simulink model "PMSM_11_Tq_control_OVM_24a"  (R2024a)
settings: Solver=VariableStepAuto  StartTime=0.0  StopTime=0.1  MaxStep=1e-6  RelTol=1e-6  AbsTol=1e-6
libraries: spsIGBTDiodeLib x6, spsVoltageMeasurementLib x4, spsCurrentMeasurementLib x3, spsControlledVoltageSourceLib x3, slpidlib x2, spsDCVoltageSourceLib x1, spsGroundLib x1, simulink x1, spsThreePhaseSeriesRLCBranchLib x1, spspowerguiLib x1

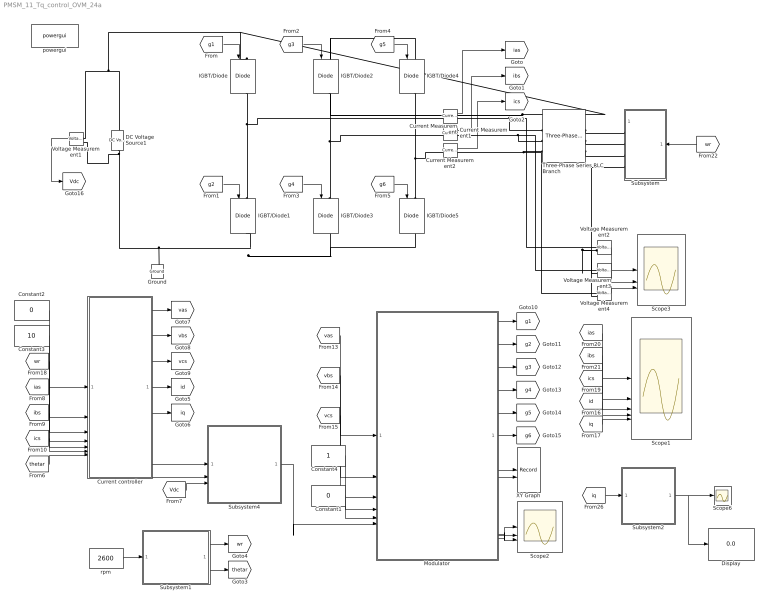
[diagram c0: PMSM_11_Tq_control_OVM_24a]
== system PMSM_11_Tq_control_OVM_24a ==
  Constant1 : Constant  Value=0
  Constant2 : Constant  Value=0
  Constant3 : Constant  Value=10
  Constant4 : Constant
  Current Measurement : spsCurrentMeasurementLib/Current Measurement  PhasorSimulation=off  OutputType=Complex  PSBequivalent=0
  Current Measurement1 : spsCurrentMeasurementLib/Current Measurement  PhasorSimulation=off  OutputType=Complex  PSBequivalent=0
  Current Measurement2 : spsCurrentMeasurementLib/Current Measurement  PhasorSimulation=off  OutputType=Complex  PSBequivalent=0
  Current controller : Subsystem
  DC Voltage Source1 : spsDCVoltageSourceLib/DC Voltage Source  Amplitude=200  Measurements=None
  Display : Display
  Ground : spsGroundLib/Ground  LConnTagsString=a
  IGBT/Diode{,1..5} (6 alike) : spsIGBTDiodeLib/IGBT//Diode  Ron=1e-3  Rs=1e5  Cs=inf  Measurements=on
  Modulator : Subsystem
  Scope1 : Scope  NumInputPorts=5
  Scope2 : Scope  NumInputPorts=3
  Scope3 : Scope  NumInputPorts=3
  Scope6 : Scope
  Subsystem : Subsystem
  Subsystem1 : Subsystem
  Subsystem2 : Subsystem
  Subsystem4 : Subsystem
  Three-Phase Series RLC Branch : spsThreePhaseSeriesRLCBranchLib/Three-Phase Series RLC Branch  LConnTagsString=A|B|C  RConnTagsString=A|B|C  BranchType=RL  Resistance=1  Inductance=2e-3  Capacitance=1e-6  Measurements=None
  Voltage Measurement{1..4} (4 alike) : spsVoltageMeasurementLib/Voltage Measurement  PhasorSimulation=off  OutputType=Complex  PSBequivalent=0
  XY Graph : Record  FileSettingsInternal="{\"entries\":[{\"content\":{\"excelSettings\":{\"content\":{},\"type\":\"Streamout.ExcelSettings\"},\"parquetSettings\":{\"content\":{},\"type\":\"Streamout.ParquetSettings\"}},\"type\":\"Streamout.FileSettingStorage\",\"uuid\":\"\"}],\"packageUris\":[\"http:\\/\\/schema.mathworks.com\\/mf0\\/streamout_blocks\\/R2020a\"],\"version\":\"1.0\"}"  Layout=[1 1]  SignalsInternal="{\"entries\":[{\"content\":{\"signals\":[{\"content\":{\"blockPath\":[],\"dimensions\":[1],\"domain\":\"\",\"lineColor\":\"#a2142f\",\"plots\":[ 1 ],\"port\":1,\"signalID\":1,\"signalName\":\"Modulator:7\"},\"type\":\"RecordBlkView.Signal\",\"uuid\":\"\"},{\"content\":{\"blockPath\":[],\"dimensions\":[1],\"domain\":\"\",\"lineColor\":\"#139fff\",\"plots\":[ 1 ],\"port\":2,\"signalID\":2,\"signalName\":\"Modulator:8\"},\"type\":\"RecordBlkView.Signal\",\"uuid\":\"\"}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"  VisualizationBindings="{\"xyplotplugin\":{\"info\":[{\"series\":[{\"bindingParametersList\":[{\"parameter\":\"X-Axis\",\"signalID\":1,\"signalName\":\"Modulator:7\"},{\"parameter\":\"Y-Axis\",\"signalID\":2,\"signalName\":\"Modulator:8\"}],\"seriesID\":0}],\"subplotID\":1}]}}"  CompatibilityTag=XY  st=0.0001
  powergui : spspowerguiLib/powergui  Priority=1  SimulationMode=Continuous  SampleTime=50e-6  frequency=60  Iterations=50  frequencyindice=0  Pbase=100e6  ErrMax=1e-4  UnitsV=kV  UnitsW=MW  buscounter=0  FunctionMessages=off  echomessages=off  EnableUseOfTLC=off  CurrentSourceSwitches=off  DisableSnubberDevices=off  DisableRonSwitches=off  DisableVfSwitches=off  DisplayEquations=off  AutomaticDiscreteSolvers=off  SolverType=Tustin/Backward Euler (TBE)  Interpol=off  ExternalGateDelay=off  methode=off  Ts=100  x0status=blocks  SPID=on  SwTol=0  HookPort=off  NonlinearTolerance=1e-4  nMaxIteration=100  ContinueOnMaxIteration=off  RestoreLinks=warning  ResistiveCurrentMeasurement=off  Frange=[0:2:500]  Ylog=off  Xlog=on  ShowGrid=off  save=off  variable=ZData  structure=0  ZoomFFT=off  StartTime=0.0  cycles=1  DisplayStyle=1  fundamental=60  FreqAxis=off  MaxFrequency=1000  frequencyindicesteady=1  RmsSteady=1  display=off
  rpm : Constant  Value=2600
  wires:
  [g1] -> IGBT/Diode/1
  [g2] -> IGBT/Diode1/1
  [g3] -> IGBT/Diode2/1
  [g4] -> IGBT/Diode3/1
  [g5] -> IGBT/Diode4/1
  [g6] -> IGBT/Diode5/1
  Current Measurement/1 -> [ias]
  Current Measurement1/1 -> [ibs]
  Current Measurement2/1 -> [ics]
  [id] -> Scope1/4
  [iq] -> Scope1/5
  [ias] -> Scope1/1
  [ics] -> Scope1/3
  [ibs] -> Scope1/2
  Voltage Measurement1/1 -> [Vdc]
  Voltage Measurement2/1 -> Scope3/1
  Voltage Measurement3/1 -> Scope3/2
  Voltage Measurement4/1 -> Scope3/3
  [wr] -> Subsystem/1(wr)
  Constant2/1 -> Current controller/1(id_ref)
  Constant3/1 -> Current controller/2(iq_ref)
  [wr] -> Current controller/3(wr)
  [ias] -> Current controller/4(ias)
  [ibs] -> Current controller/5(ibs)
  [ics] -> Current controller/6(ics)
  Current controller/1(vas) -> [vas]
  Current controller/2(vbs) -> [vbs]
  Current controller/3(vcs) -> [vcs]
  [thetar] -> Current controller/7(thetar)
  Current controller/4(id) -> [id]
  Current controller/5(iq) -> [iq]
  rpm/1 -> Subsystem1/1(rpm_ref)
  Subsystem1/1(wr) -> [wr]
  Subsystem1/2(thetar) -> [thetar]
  [vas] -> Modulator/1(vas)
  [vbs] -> Modulator/2(vbs)
  [vcs] -> Modulator/3(vcs)
  Constant4/1 -> Modulator/4(SVM_MODE)
  Constant1/1 -> Modulator/5(OVMgain)
  Modulator/1(g1) -> [g1]
  Modulator/2(g2) -> [g2]
  Modulator/3(g3) -> [g3]
  Modulator/4(g4) -> [g4]
  Modulator/5(g5) -> [g5]
  Modulator/6(g6) -> [g6]
  Subsystem2/1(Tq_avg) -> Scope6/1, Display/1
  [iq] -> Subsystem2/1(Iq)
  Modulator/7(Vds) -> XY Graph/1
  Modulator/8(Vqs) -> XY Graph/2
  Modulator/9(Van) -> Scope2/1
  Modulator/10(Vbn) -> Scope2/2
  Modulator/11(Vcn) -> Scope2/3
  Current controller/6(vds) -> Subsystem4/1(Vds)
  Current controller/7(vqs) -> Subsystem4/2(Vqs)
  [Vdc] -> Subsystem4/3(Vdc)
  Subsystem4/1(Flag_OVM) -> Modulator/6(Flag_OVM)
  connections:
  IGBT/Diode1/LConn1 -- Current Measurement/LConn1 -- IGBT/Diode/RConn1
  Voltage Measurement1/LConn1 -- IGBT/Diode4/LConn1 -- IGBT/Diode2/LConn1 -- IGBT/Diode/LConn1 -- DC Voltage Source1/RConn1
  DC Voltage Source1/LConn1 -- Voltage Measurement1/LConn2 -- IGBT/Diode3/RConn1 -- IGBT/Diode5/RConn1 -- IGBT/Diode1/RConn1 -- Ground/LConn1
  IGBT/Diode3/LConn1 -- Current Measurement1/LConn1 -- IGBT/Diode2/RConn1
  IGBT/Diode5/LConn1 -- Current Measurement2/LConn1 -- IGBT/Diode4/RConn1
  Three-Phase Series RLC Branch/RConn1 -- Subsystem/RConn1
  Three-Phase Series RLC Branch/RConn2 -- Subsystem/RConn2
  Three-Phase Series RLC Branch/RConn3 -- Subsystem/RConn3
  Current Measurement/RConn1 -- Voltage Measurement2/LConn1 -- Three-Phase Series RLC Branch/LConn1
  Current Measurement1/RConn1 -- Voltage Measurement3/LConn1 -- Three-Phase Series RLC Branch/LConn2
  Current Measurement2/RConn1 -- Voltage Measurement4/LConn1 -- Three-Phase Series RLC Branch/LConn3
  Voltage Measurement2/LConn2 -- Voltage Measurement4/LConn2 -- Voltage Measurement3/LConn2 -- Subsystem/RConn4

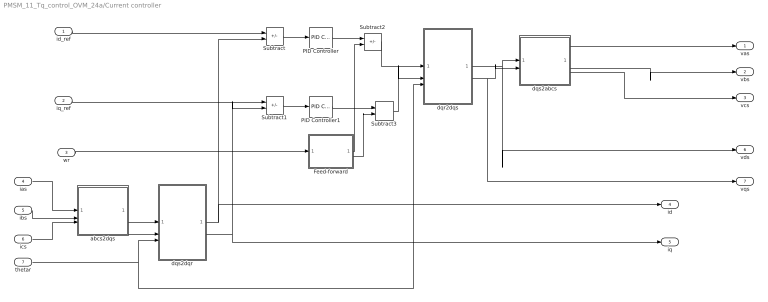
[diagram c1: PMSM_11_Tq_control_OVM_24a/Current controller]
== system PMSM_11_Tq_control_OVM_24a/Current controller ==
  id_ref : Inport
  iq_ref : Inport  Port=2
  wr : Inport  Port=3
  ias : Inport  Port=4
  ibs : Inport  Port=5
  ics : Inport  Port=6
  thetar : Inport  Port=7
  Feed-forward : Subsystem
  PID Controller : slpidlib/PID Controller  Controller=PI  Form=Parallel  TimeDomain=Continuous-time  UseExternalTs=off  SampleTime=-1  IntegratorMethod=Forward Euler  FilterMethod=Forward Euler  ControllerParametersSource=internal  P=2*pi*300*0.002  I=2*pi*300*1  UseKiTs=off  D=0  UseExternalDerivativeSource=off  N=100  UseFilter=on  TunerSelectOption=Transfer Function Based (PID Tuner App)  InitialConditionSource=internal  InitialConditionForIntegrator=0  InitialConditionForFilter=0  DifferentiatorICPrevScaledInput=0  ExternalReset=none  TrackingMode=off  Kt=1  LimitOutput=off  SatLimitsSource=internal  UpperSaturationLimit=inf  LowerSaturationLimit=-inf  LinearizeAsGain=on  AntiWindupMode=none  Kb=1  LimitIntegrator=off  UpperIntegratorSaturationLimit=inf  LowerIntegratorSaturationLimit=-inf  POutMin=[]  POutMax=[]  IOutMin=[]  IOutMax=[]  DOutMin=[]  DOutMax=[]  NOutMin=[]  NOutMax=[]  SumOutMin=[]  SumOutMax=[]  SaturationOutMin=[]  SaturationOutMax=[]  PParamMin=[]  PParamMax=[]  IParamMin=[]  IParamMax=[]  DParamMin=[]  DParamMax=[]  NParamMin=[]  NParamMax=[]  KbParamMin=[]  KbParamMax=[]  KtParamMin=[]  KtParamMax=[]  KbOutMin=[]  KbOutMax=[]  KtOutMin=[]  KtOutMax=[]  IntegratorOutMin=[]  IntegratorOutMax=[]  FilterOutMin=[]  FilterOutMax=[]  SumI1OutMin=[]  SumI1OutMax=[]  SumI2OutMin=[]  SumI2OutMax=[]  SumI3OutMin=[]  SumI3OutMax=[]  SumI4OutMin=[]  SumI4OutMax=[]  SumDOutMin=[]  SumDOutMax=[]  DifferentiatorOutMin=[]  DifferentiatorOutMax=[]  FilterDiffOutCoefMin=[]  FilterDiffOutCoefMax=[]  ReciprocalOutMin=[]  ReciprocalOutMax=[]  SumDenOutMin=[]  SumDenOutMax=[]  SumNumOutMin=[]  SumNumOutMax=[]  DivideOutMin=[]  DivideOutMax=[]  UdiffTsProdOutMin=[]  UdiffTsProdOutMax=[]  NTsProdOutMin=[]  NTsProdOutMax=[]  UintegralTsProdOutMin=[]  UintegralTsProdOutMax=[]  UngainTsProdOutMin=[]  UngainTsProdOutMax=[]  ClampingZeroOutDataTypeStr=Inherit: Inherit via back propagation  ClampingZeroOutMin=[]  ClampingZeroOutMax=[]  FilterDenConstantOutDataTypeStr=Inherit: Inherit via back propagation  FilterDenConstantOutMin=[]  FilterDenConstantOutMax=[]  PCopyOutDataTypeStr=Inherit: Inherit via back propagation  PCopyOutMin=[]  PCopyOutMax=[]  NCopyOutDataTypeStr=Inherit: Inherit via back propagation  NCopyOutMin=[]  NCopyOutMax=[]  IntegratorContinuousStateAttributes=''  IntegratorStateMustResolveToSignalObject=off  IntegratorRTWStateStorageClass=Auto  FilterContinuousStateAttributes=''  FilterStateMustResolveToSignalObject=off  FilterRTWStateStorageClass=Auto  ParallelPVariant=InternalParameters  IdealPVariant=Disabled  IVariant=InternalParameters  DVariant=Disabled  IntegratorVariant=Continuous  SatVariant=Disabled  AWVariant=Passthrough  PCopyVariant=Disabled  TRVariant=Disabled  FdbkBlocksVariant=Forward  IdealPFdbkVariant=Disabled  SatFdbkVariant=Disabled  DerivativeFilterVariant=Disabled  NVariant=Disabled  NCopyVariant=Disabled_SignalSpec  FilterICVariant=Disabled  IntegratorICVariant=InternalICs  ExternalResetVariant=Disabled  TRSumVariant=Passthrough  SumFdbkVariant=Disabled  SumVariant=Sum_PI  TsampFilterVariant=InternalTs  TsampNgainVariant=Passthrough  TsampIntegralVariant=Disabled_SignalSpec  ExternalSaturationOutDataTypeStr=Inherit: Same as second input  DerivativeSourceVariant=Disabled
  PID Controller1 : slpidlib/PID Controller  Controller=PI  Form=Parallel  TimeDomain=Continuous-time  UseExternalTs=off  SampleTime=-1  IntegratorMethod=Forward Euler  FilterMethod=Forward Euler  ControllerParametersSource=internal  P=2*pi*300*0.002  I=2*pi*300*1  UseKiTs=off  D=0  UseExternalDerivativeSource=off  N=100  UseFilter=on  TunerSelectOption=Transfer Function Based (PID Tuner App)  InitialConditionSource=internal  InitialConditionForIntegrator=0  InitialConditionForFilter=0  DifferentiatorICPrevScaledInput=0  ExternalReset=none  TrackingMode=off  Kt=1  LimitOutput=off  SatLimitsSource=internal  UpperSaturationLimit=inf  LowerSaturationLimit=-inf  LinearizeAsGain=on  AntiWindupMode=none  Kb=1  LimitIntegrator=off  UpperIntegratorSaturationLimit=inf  LowerIntegratorSaturationLimit=-inf  POutMin=[]  POutMax=[]  IOutMin=[]  IOutMax=[]  DOutMin=[]  DOutMax=[]  NOutMin=[]  NOutMax=[]  SumOutMin=[]  SumOutMax=[]  SaturationOutMin=[]  SaturationOutMax=[]  PParamMin=[]  PParamMax=[]  IParamMin=[]  IParamMax=[]  DParamMin=[]  DParamMax=[]  NParamMin=[]  NParamMax=[]  KbParamMin=[]  KbParamMax=[]  KtParamMin=[]  KtParamMax=[]  KbOutMin=[]  KbOutMax=[]  KtOutMin=[]  KtOutMax=[]  IntegratorOutMin=[]  IntegratorOutMax=[]  FilterOutMin=[]  FilterOutMax=[]  SumI1OutMin=[]  SumI1OutMax=[]  SumI2OutMin=[]  SumI2OutMax=[]  SumI3OutMin=[]  SumI3OutMax=[]  SumI4OutMin=[]  SumI4OutMax=[]  SumDOutMin=[]  SumDOutMax=[]  DifferentiatorOutMin=[]  DifferentiatorOutMax=[]  FilterDiffOutCoefMin=[]  FilterDiffOutCoefMax=[]  ReciprocalOutMin=[]  ReciprocalOutMax=[]  SumDenOutMin=[]  SumDenOutMax=[]  SumNumOutMin=[]  SumNumOutMax=[]  DivideOutMin=[]  DivideOutMax=[]  UdiffTsProdOutMin=[]  UdiffTsProdOutMax=[]  NTsProdOutMin=[]  NTsProdOutMax=[]  UintegralTsProdOutMin=[]  UintegralTsProdOutMax=[]  UngainTsProdOutMin=[]  UngainTsProdOutMax=[]  ClampingZeroOutDataTypeStr=Inherit: Inherit via back propagation  ClampingZeroOutMin=[]  ClampingZeroOutMax=[]  FilterDenConstantOutDataTypeStr=Inherit: Inherit via back propagation  FilterDenConstantOutMin=[]  FilterDenConstantOutMax=[]  PCopyOutDataTypeStr=Inherit: Inherit via back propagation  PCopyOutMin=[]  PCopyOutMax=[]  NCopyOutDataTypeStr=Inherit: Inherit via back propagation  NCopyOutMin=[]  NCopyOutMax=[]  IntegratorContinuousStateAttributes=''  IntegratorStateMustResolveToSignalObject=off  IntegratorRTWStateStorageClass=Auto  FilterContinuousStateAttributes=''  FilterStateMustResolveToSignalObject=off  FilterRTWStateStorageClass=Auto  ParallelPVariant=InternalParameters  IdealPVariant=Disabled  IVariant=InternalParameters  DVariant=Disabled  IntegratorVariant=Continuous  SatVariant=Disabled  AWVariant=Passthrough  PCopyVariant=Disabled  TRVariant=Disabled  FdbkBlocksVariant=Forward  IdealPFdbkVariant=Disabled  SatFdbkVariant=Disabled  DerivativeFilterVariant=Disabled  NVariant=Disabled  NCopyVariant=Disabled_SignalSpec  FilterICVariant=Disabled  IntegratorICVariant=InternalICs  ExternalResetVariant=Disabled  TRSumVariant=Passthrough  SumFdbkVariant=Disabled  SumVariant=Sum_PI  TsampFilterVariant=InternalTs  TsampNgainVariant=Passthrough  TsampIntegralVariant=Disabled_SignalSpec  ExternalSaturationOutDataTypeStr=Inherit: Same as second input  DerivativeSourceVariant=Disabled
  Subtract : Sum  Inputs=+-
  Subtract1 : Sum  Inputs=+-
  Subtract2 : Sum  Inputs=+-
  Subtract3 : Sum
  abcs2dqs : Subsystem
  dqr2dqs : Subsystem
  dqs2abcs : Subsystem
  dqs2dqr : Subsystem
  vas : Outport  VectorParamsAs1DForOutWhenUnconnected=off
  vbs : Outport  Port=2  VectorParamsAs1DForOutWhenUnconnected=off
  vcs : Outport  Port=3  VectorParamsAs1DForOutWhenUnconnected=off
  id : Outport  Port=4  VectorParamsAs1DForOutWhenUnconnected=off
  iq : Outport  Port=5  VectorParamsAs1DForOutWhenUnconnected=off
  vds : Outport  Port=6  VectorParamsAs1DForOutWhenUnconnected=off
  vqs : Outport  Port=7  VectorParamsAs1DForOutWhenUnconnected=off
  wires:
  thetar/1 -> dqs2dqr/3(thetar), dqr2dqs/3(thetar)
  dqr2dqs/2(qs) -> vqs/1, dqs2abcs/2(qs)
  dqr2dqs/1(ds) -> vds/1, dqs2abcs/1(ds)
  dqs2dqr/1(dr) -> id/1, Subtract/2
  abcs2dqs/1(ds) -> dqs2dqr/1(ds)
  Subtract/1 -> PID Controller/1
  dqs2dqr/2(qr) -> Subtract1/2, iq/1
  Subtract1/1 -> PID Controller1/1
  Feed-forward/1(Edr) -> Subtract2/2
  PID Controller1/1 -> Subtract3/1
  Subtract3/1 -> dqr2dqs/2(qr)
  abcs2dqs/2(qs) -> dqs2dqr/2(qs)
  ics/1 -> abcs2dqs/3(cs)
  Subtract2/1 -> dqr2dqs/1(dr)
  Feed-forward/2(Eqr) -> Subtract3/2
  PID Controller/1 -> Subtract2/1
  wr/1 -> Feed-forward/1(wr)
  iq_ref/1 -> Subtract1/1
  id_ref/1 -> Subtract/1
  ibs/1 -> abcs2dqs/2(bs)
  ias/1 -> abcs2dqs/1(as)
  dqs2abcs/1(as) -> vas/1
  dqs2abcs/2(bs) -> vbs/1
  dqs2abcs/3(cs) -> vcs/1

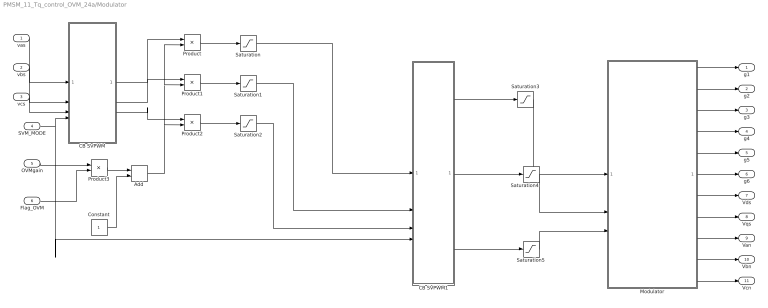
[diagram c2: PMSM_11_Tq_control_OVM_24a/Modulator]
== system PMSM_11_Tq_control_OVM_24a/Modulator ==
  vas : Inport
  vbs : Inport  Port=2
  vcs : Inport  Port=3
  SVM_MODE : Inport  Port=4
  OVMgain : Inport  Port=5
  Flag_OVM : Inport  Port=6
  Add : Sum
  CB SVPWM : Subsystem
  CB SVPWM1 : Subsystem
  Constant : Constant
  Modulator : Subsystem
  Product{,1..3} (4 alike) : Product
  Saturation{,1..5} (6 alike) : Saturate  UpperLimit=100  LowerLimit=-100
  g1 : Outport  VectorParamsAs1DForOutWhenUnconnected=off
  g2 : Outport  Port=2  VectorParamsAs1DForOutWhenUnconnected=off
  g3 : Outport  Port=3  VectorParamsAs1DForOutWhenUnconnected=off
  g4 : Outport  Port=4  VectorParamsAs1DForOutWhenUnconnected=off
  g5 : Outport  Port=5  VectorParamsAs1DForOutWhenUnconnected=off
  g6 : Outport  Port=6  VectorParamsAs1DForOutWhenUnconnected=off
  Vds : Outport  Port=7  VectorParamsAs1DForOutWhenUnconnected=off
  Vqs : Outport  Port=8  VectorParamsAs1DForOutWhenUnconnected=off
  Van : Outport  Port=9  VectorParamsAs1DForOutWhenUnconnected=off
  Vbn : Outport  Port=10  VectorParamsAs1DForOutWhenUnconnected=off
  Vcn : Outport  Port=11  VectorParamsAs1DForOutWhenUnconnected=off
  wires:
  CB SVPWM1/3(vcn) -> Saturation5/1
  vcs/1 -> CB SVPWM/3(vcs)
  Modulator/2(g2) -> g2/1
  CB SVPWM1/1(van) -> Saturation3/1
  Modulator/9(Van_inv) -> Van/1
  CB SVPWM1/2(vbn) -> Saturation4/1
  Modulator/5(g5) -> g5/1
  Modulator/4(g4) -> g4/1
  SVM_MODE/1 -> CB SVPWM1/4(SVM), CB SVPWM/4(SVM)
  vbs/1 -> CB SVPWM/2(vbs)
  Modulator/1(g1) -> g1/1
  Modulator/8(Vqs_stator) -> Vqs/1
  Modulator/6(g6) -> g6/1
  vas/1 -> CB SVPWM/1(vas)
  Modulator/10(Vbn_inv) -> Vbn/1
  Modulator/11(Vcn_inv) -> Vcn/1
  Modulator/7(Vds_stator) -> Vds/1
  Modulator/3(g3) -> g3/1
  Saturation3/1 -> Modulator/1(van)
  Saturation4/1 -> Modulator/2(vbn)
  Saturation5/1 -> Modulator/3(vcn)
  Product/1 -> Saturation/1
  Product1/1 -> Saturation1/1
  Product2/1 -> Saturation2/1
  CB SVPWM/1(van) -> Product/1
  CB SVPWM/3(vcn) -> Product2/1
  CB SVPWM/2(vbn) -> Product1/1
  OVMgain/1 -> Product3/1
  Flag_OVM/1 -> Product3/2
  Product3/1 -> Add/1
  Add/1 -> Product2/2, Product1/2, Product/2
  Constant/1 -> Add/2
  Saturation/1 -> CB SVPWM1/1(vas)
  Saturation1/1 -> CB SVPWM1/2(vbs)
  Saturation2/1 -> CB SVPWM1/3(vcs)

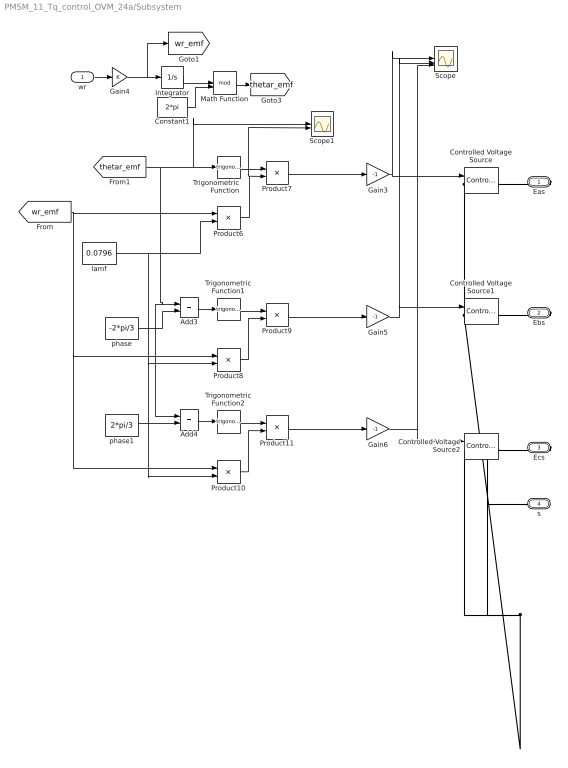
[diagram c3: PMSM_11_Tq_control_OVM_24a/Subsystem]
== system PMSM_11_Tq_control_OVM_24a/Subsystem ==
  wr : Inport
  Add3 : Sum
  Add4 : Sum
  Constant1 : Constant  Value=2*pi
  Controlled Voltage Source : spsControlledVoltageSourceLib/Controlled Voltage Source  Initialize=on  Source_Type=AC  Amplitude=0  Phase=0  Frequency=0  Measurements=None
  Controlled Voltage Source1 : spsControlledVoltageSourceLib/Controlled Voltage Source  Initialize=on  Source_Type=AC  Amplitude=0  Phase=0  Frequency=0  Measurements=None
  Controlled Voltage Source2 : spsControlledVoltageSourceLib/Controlled Voltage Source  Initialize=on  Source_Type=AC  Amplitude=0  Phase=0  Frequency=0  Measurements=None
  Gain3 : Gain  Gain=-1
  Gain4 : Gain
  Gain5 : Gain  Gain=-1
  Gain6 : Gain  Gain=-1
  Integrator : Integrator
  Math Function : Math  Operator=mod  SignedPower=on
  Product{6..11} (6 alike) : Product
  Scope : Scope  NumInputPorts=3
  Scope1 : Scope  NumInputPorts=2
  Trigonometric Function : Trigonometry
  Trigonometric Function1 : Trigonometry
  Trigonometric Function2 : Trigonometry
  lamf : Constant  Value=0.0796
  phase : Constant  Value=-2*pi/3
  phase1 : Constant  Value=2*pi/3
  Eas : PMIOPort  Side=Right
  Ebs : PMIOPort  Port=2  Side=Right
  Ecs : PMIOPort  Port=3  Side=Right
  s : PMIOPort  Port=4  Side=Right
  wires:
  Integrator/1 -> Math Function/1
  Constant1/1 -> Math Function/2
  Math Function/1 -> [thetar_emf]
  wr/1 -> Gain4/1
  Trigonometric Function/1 -> Product7/1
  Product6/1 -> Scope1/2, Product7/2
  Gain4/1 -> [wr_emf], Integrator/1
  Product7/1 -> Gain3/1
  Product9/1 -> Gain5/1
  Product8/1 -> Product9/2
  Trigonometric Function1/1 -> Product9/1
  [thetar_emf] -> Add4/1, Add3/1, Scope1/1, Trigonometric Function/1
  Add3/1 -> Trigonometric Function1/1
  phase/1 -> Add3/2
  Gain5/1 -> Controlled Voltage Source1/1, Scope/2
  Gain3/1 -> Controlled Voltage Source/1, Scope/1
  phase1/1 -> Add4/2
  Add4/1 -> Trigonometric Function2/1
  [wr_emf] -> Product10/1, Product8/1, Product6/1
  Trigonometric Function2/1 -> Product11/1
  Product10/1 -> Product11/2
  Product11/1 -> Gain6/1
  lamf/1 -> Product8/2, Product10/2, Product6/2
  Gain6/1 -> Controlled Voltage Source2/1, Scope/3
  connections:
  Eas/RConn1 -- Controlled Voltage Source/RConn1
  Ebs/RConn1 -- Controlled Voltage Source1/RConn1
  Ecs/RConn1 -- Controlled Voltage Source2/RConn1
  Controlled Voltage Source/LConn1 -- s/RConn1 -- Controlled Voltage Source2/LConn1 -- Controlled Voltage Source1/LConn1

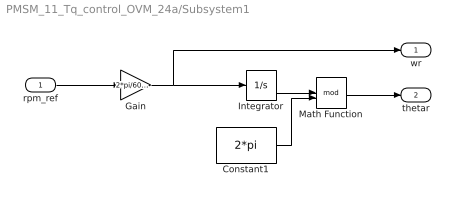
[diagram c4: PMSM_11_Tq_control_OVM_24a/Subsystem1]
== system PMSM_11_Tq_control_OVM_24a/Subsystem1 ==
  rpm_ref : Inport
  Constant1 : Constant  Value=2*pi
  Gain : Gain  Gain=2*pi/60*4
  Integrator : Integrator
  Math Function : Math  Operator=mod  SignedPower=on
  wr : Outport  VectorParamsAs1DForOutWhenUnconnected=off
  thetar : Outport  Port=2  VectorParamsAs1DForOutWhenUnconnected=off
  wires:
  Math Function/1 -> thetar/1
  Integrator/1 -> Math Function/1
  Gain/1 -> wr/1, Integrator/1
  rpm_ref/1 -> Gain/1
  Constant1/1 -> Math Function/2

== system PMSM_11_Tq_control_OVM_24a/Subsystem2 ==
  Iq : Inport
  Tq_constant : Gain  Gain=3/4*4*0.0796
  Transfer Fcn : TransferFcn  Numerator=[2*pi*50]  Denominator=[1 2*pi*50]
  Tq_avg : Outport  VectorParamsAs1DForOutWhenUnconnected=off
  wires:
  Transfer Fcn/1 -> Tq_avg/1
  Iq/1 -> Tq_constant/1
  Tq_constant/1 -> Transfer Fcn/1

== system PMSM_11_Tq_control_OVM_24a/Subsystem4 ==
  Vds : Inport
  Vqs : Inport  Port=2
  Vdc : Inport  Port=3
  Gain : Gain  Gain=1/sqrt(3)
  Relational Operator : RelationalOperator  Operator=>  OutDataTypeStr=boolean  RndMeth=Simplest
  Subsystem3 : Subsystem
  Flag_OVM : Outport
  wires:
  Subsystem3/1(Out1) -> Relational Operator/1
  Vdc/1 -> Gain/1
  Relational Operator/1 -> Flag_OVM/1
  Vds/1 -> Subsystem3/1(In1)
  Gain/1 -> Relational Operator/2
  Vqs/1 -> Subsystem3/2(In2)

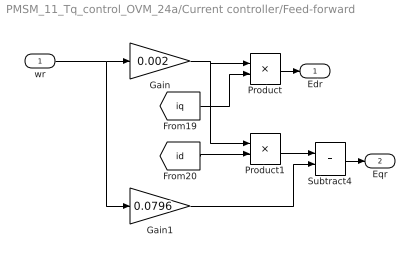
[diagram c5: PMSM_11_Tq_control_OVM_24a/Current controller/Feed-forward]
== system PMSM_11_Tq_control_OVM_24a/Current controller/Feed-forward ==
  wr : Inport
  Gain : Gain  Gain=0.002
  Gain1 : Gain  Gain=0.0796
  Product : Product
  Product1 : Product
  Subtract4 : Sum
  Edr : Outport  VectorParamsAs1DForOutWhenUnconnected=off
  Eqr : Outport  Port=2  VectorParamsAs1DForOutWhenUnconnected=off
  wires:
  Gain/1 -> Product1/1, Product/1
  Gain1/1 -> Subtract4/2
  [id] -> Product1/2
  wr/1 -> Gain1/1, Gain/1
  Product1/1 -> Subtract4/1
  [iq] -> Product/2
  Product/1 -> Edr/1
  Subtract4/1 -> Eqr/1

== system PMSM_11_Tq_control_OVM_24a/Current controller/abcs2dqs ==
  as : Inport
  bs : Inport  Port=2
  cs : Inport  Port=3
  Gain : Gain  Gain=1/sqrt(3)
  Subtract : Sum  Inputs=+-
  ds : Outport  VectorParamsAs1DForOutWhenUnconnected=off
  qs : Outport  Port=2  VectorParamsAs1DForOutWhenUnconnected=off
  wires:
  Subtract/1 -> Gain/1
  Gain/1 -> qs/1
  bs/1 -> Subtract/1
  cs/1 -> Subtract/2
  as/1 -> ds/1

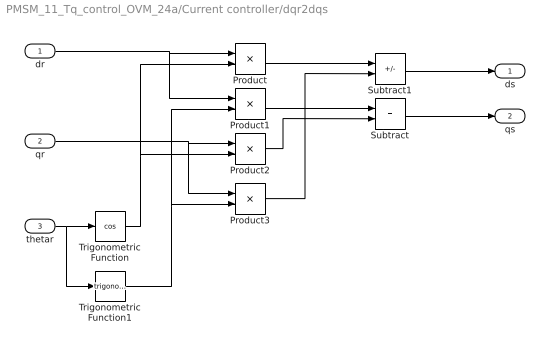
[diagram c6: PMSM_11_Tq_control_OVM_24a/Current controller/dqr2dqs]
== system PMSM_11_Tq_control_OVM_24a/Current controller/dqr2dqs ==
  dr : Inport
  qr : Inport  Port=2
  thetar : Inport  Port=3
  Product{,1..3} (4 alike) : Product
  Subtract : Sum
  Subtract1 : Sum  Inputs=+-
  Trigonometric Function : Trigonometry  Operator=cos
  Trigonometric Function1 : Trigonometry
  ds : Outport  VectorParamsAs1DForOutWhenUnconnected=off
  qs : Outport  Port=2  VectorParamsAs1DForOutWhenUnconnected=off
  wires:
  Subtract1/1 -> ds/1
  Product2/1 -> Subtract/2
  Product1/1 -> Subtract/1
  Product3/1 -> Subtract1/2
  Product/1 -> Subtract1/1
  qr/1 -> Product2/1, Product3/1
  Trigonometric Function1/1 -> Product1/2, Product3/2
  Trigonometric Function/1 -> Product/2, Product2/2
  dr/1 -> Product/1, Product1/1
  thetar/1 -> Trigonometric Function/1, Trigonometric Function1/1
  Subtract/1 -> qs/1

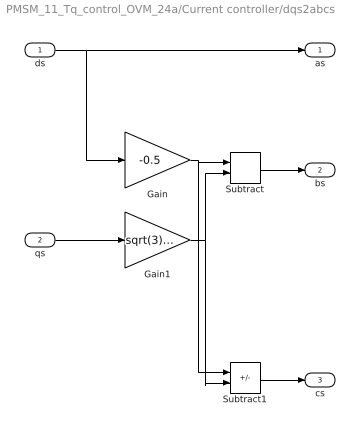
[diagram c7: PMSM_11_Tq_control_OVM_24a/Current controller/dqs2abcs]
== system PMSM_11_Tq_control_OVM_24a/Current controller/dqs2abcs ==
  ds : Inport
  qs : Inport  Port=2
  Gain : Gain  Gain=-0.5
  Gain1 : Gain  Gain=sqrt(3)/2
  Subtract : Sum
  Subtract1 : Sum  Inputs=+-
  as : Outport  VectorParamsAs1DForOutWhenUnconnected=off
  bs : Outport  Port=2  VectorParamsAs1DForOutWhenUnconnected=off
  cs : Outport  Port=3  VectorParamsAs1DForOutWhenUnconnected=off
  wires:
  ds/1 -> Gain/1, as/1
  Gain/1 -> Subtract1/1, Subtract/1
  qs/1 -> Gain1/1
  Gain1/1 -> Subtract/2, Subtract1/2
  Subtract/1 -> bs/1
  Subtract1/1 -> cs/1

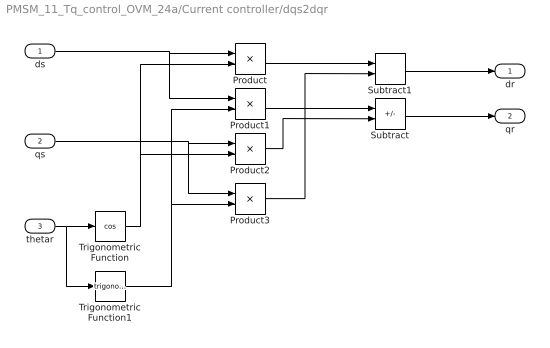
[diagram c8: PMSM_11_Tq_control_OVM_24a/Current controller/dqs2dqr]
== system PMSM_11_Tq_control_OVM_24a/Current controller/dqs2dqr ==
  ds : Inport
  qs : Inport  Port=2
  thetar : Inport  Port=3
  Product{,1..3} (4 alike) : Product
  Subtract : Sum  Inputs=-+
  Subtract1 : Sum
  Trigonometric Function : Trigonometry  Operator=cos
  Trigonometric Function1 : Trigonometry
  dr : Outport  VectorParamsAs1DForOutWhenUnconnected=off
  qr : Outport  Port=2  VectorParamsAs1DForOutWhenUnconnected=off
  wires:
  Subtract/1 -> qr/1
  thetar/1 -> Trigonometric Function1/1, Trigonometric Function/1
  ds/1 -> Product1/1, Product/1
  Trigonometric Function/1 -> Product2/2, Product/2
  Trigonometric Function1/1 -> Product3/2, Product1/2
  qs/1 -> Product3/1, Product2/1
  Product/1 -> Subtract1/1
  Product3/1 -> Subtract1/2
  Product1/1 -> Subtract/1
  Product2/1 -> Subtract/2
  Subtract1/1 -> dr/1

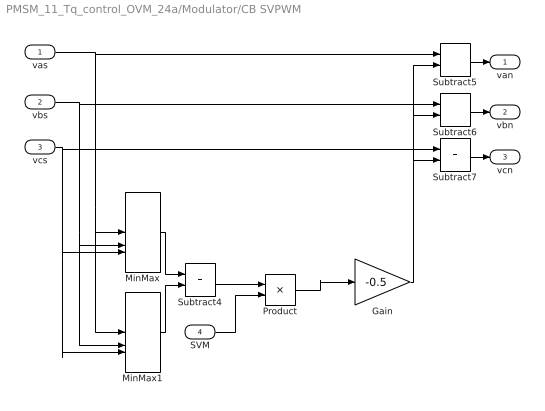
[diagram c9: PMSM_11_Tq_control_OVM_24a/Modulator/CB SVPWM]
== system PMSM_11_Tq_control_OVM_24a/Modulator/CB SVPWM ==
  vas : Inport
  vbs : Inport  Port=2
  vcs : Inport  Port=3
  SVM : Inport  Port=4
  Gain : Gain  Gain=-0.5
  MinMax : MinMax  Function=max  Inputs=3
  MinMax1 : MinMax  Inputs=3
  Product : Product
  Subtract{4..7} (4 alike) : Sum
  van : Outport  VectorParamsAs1DForOutWhenUnconnected=off
  vbn : Outport  Port=2  VectorParamsAs1DForOutWhenUnconnected=off
  vcn : Outport  Port=3  VectorParamsAs1DForOutWhenUnconnected=off
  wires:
  MinMax/1 -> Subtract4/1
  MinMax1/1 -> Subtract4/2
  vcs/1 -> MinMax1/3, MinMax/3, Subtract7/1
  Subtract6/1 -> vbn/1
  vbs/1 -> MinMax1/2, MinMax/2, Subtract6/1
  Subtract5/1 -> van/1
  Gain/1 -> Subtract6/2, Subtract5/2, Subtract7/2
  vas/1 -> MinMax1/1, MinMax/1, Subtract5/1
  Subtract7/1 -> vcn/1
  Subtract4/1 -> Product/1
  Product/1 -> Gain/1
  SVM/1 -> Product/2

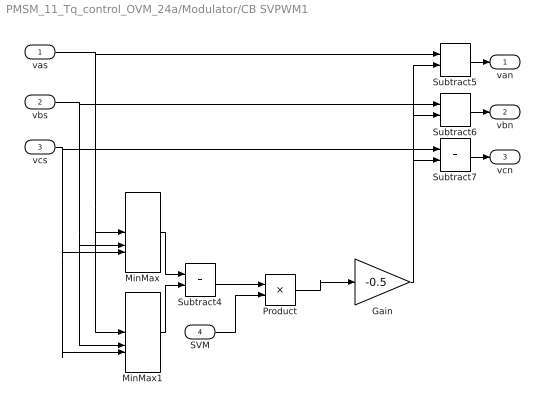
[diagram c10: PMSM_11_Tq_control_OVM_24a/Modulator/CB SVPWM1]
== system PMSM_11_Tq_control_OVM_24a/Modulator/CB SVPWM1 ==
  vas : Inport
  vbs : Inport  Port=2
  vcs : Inport  Port=3
  SVM : Inport  Port=4
  Gain : Gain  Gain=-0.5
  MinMax : MinMax  Function=max  Inputs=3
  MinMax1 : MinMax  Inputs=3
  Product : Product
  Subtract{4..7} (4 alike) : Sum
  van : Outport  VectorParamsAs1DForOutWhenUnconnected=off
  vbn : Outport  Port=2  VectorParamsAs1DForOutWhenUnconnected=off
  vcn : Outport  Port=3  VectorParamsAs1DForOutWhenUnconnected=off
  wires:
  SVM/1 -> Product/2
  Product/1 -> Gain/1
  Subtract4/1 -> Product/1
  Subtract7/1 -> vcn/1
  vas/1 -> Subtract5/1, MinMax/1, MinMax1/1
  Gain/1 -> Subtract7/2, Subtract5/2, Subtract6/2
  Subtract5/1 -> van/1
  vbs/1 -> Subtract6/1, MinMax/2, MinMax1/2
  Subtract6/1 -> vbn/1
  vcs/1 -> Subtract7/1, MinMax/3, MinMax1/3
  MinMax1/1 -> Subtract4/2
  MinMax/1 -> Subtract4/1

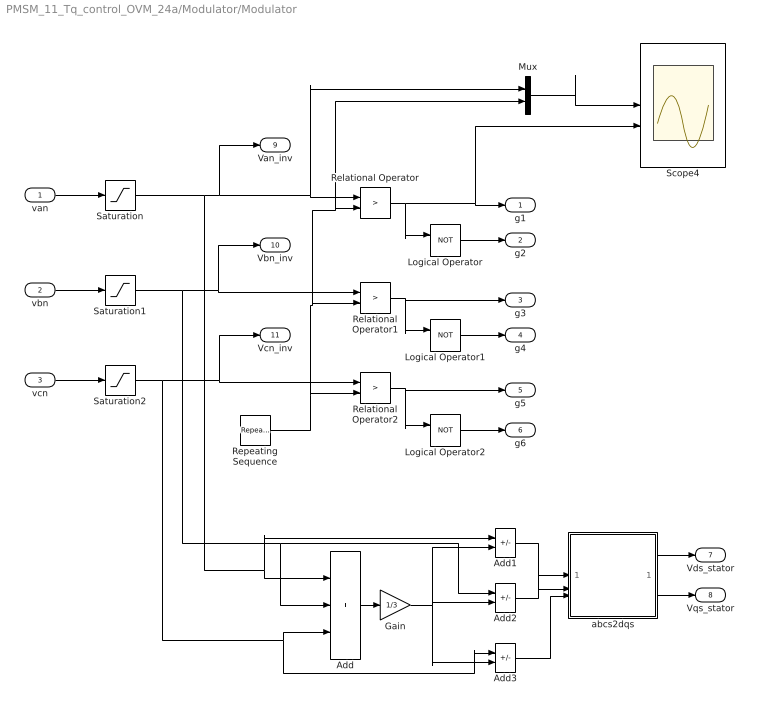
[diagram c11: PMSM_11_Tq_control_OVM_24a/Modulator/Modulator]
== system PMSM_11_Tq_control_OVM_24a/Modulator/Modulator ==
  van : Inport
  vbn : Inport  Port=2
  vcn : Inport  Port=3
  Add : Sum  Inputs=+++
  Add1 : Sum  Inputs=+-
  Add2 : Sum  Inputs=+-
  Add3 : Sum  Inputs=+-
  Gain : Gain  Gain=1/3
  Logical Operator : Logic  Operator=NOT  AllPortsSameDT=off  OutDataTypeStr=boolean
  Logical Operator1 : Logic  Operator=NOT  AllPortsSameDT=off  OutDataTypeStr=boolean
  Logical Operator2 : Logic  Operator=NOT  AllPortsSameDT=off  OutDataTypeStr=boolean
  Mux : Mux  Inputs=2
  Relational Operator : RelationalOperator  Operator=>  OutDataTypeStr=boolean  RndMeth=Simplest
  Relational Operator1 : RelationalOperator  Operator=>  OutDataTypeStr=boolean  RndMeth=Simplest
  Relational Operator2 : RelationalOperator  Operator=>  OutDataTypeStr=boolean  RndMeth=Simplest
  Repeating Sequence : simulink/Sources/Repeating Sequence  rep_seq_t=[0 0.00005 0.0001]  rep_seq_y=[-100 100 -100]
  Saturation : Saturate  UpperLimit=100  LowerLimit=-100
  Saturation1 : Saturate  UpperLimit=100  LowerLimit=-100
  Saturation2 : Saturate  UpperLimit=100  LowerLimit=-100
  Scope4 : Scope  NumInputPorts=2
  abcs2dqs : Subsystem
  g1 : Outport  VectorParamsAs1DForOutWhenUnconnected=off
  g2 : Outport  Port=2  VectorParamsAs1DForOutWhenUnconnected=off
  g3 : Outport  Port=3  VectorParamsAs1DForOutWhenUnconnected=off
  g4 : Outport  Port=4  VectorParamsAs1DForOutWhenUnconnected=off
  g5 : Outport  Port=5  VectorParamsAs1DForOutWhenUnconnected=off
  g6 : Outport  Port=6  VectorParamsAs1DForOutWhenUnconnected=off
  Vds_stator : Outport  Port=7  VectorParamsAs1DForOutWhenUnconnected=off
  Vqs_stator : Outport  Port=8  VectorParamsAs1DForOutWhenUnconnected=off
  Van_inv : Outport  Port=9  VectorParamsAs1DForOutWhenUnconnected=off
  Vbn_inv : Outport  Port=10  VectorParamsAs1DForOutWhenUnconnected=off
  Vcn_inv : Outport  Port=11  VectorParamsAs1DForOutWhenUnconnected=off
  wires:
  van/1 -> Saturation/1
  Relational Operator/1 -> Scope4/2, g1/1, Logical Operator/1
  Relational Operator1/1 -> g3/1, Logical Operator1/1
  Relational Operator2/1 -> g5/1, Logical Operator2/1
  Logical Operator1/1 -> g4/1
  Logical Operator2/1 -> g6/1
  Logical Operator/1 -> g2/1
  vbn/1 -> Saturation1/1
  vcn/1 -> Saturation2/1
  Repeating Sequence/1 -> Mux/2, Relational Operator/2, Relational Operator1/2, Relational Operator2/2
  Add2/1 -> abcs2dqs/2(bs)
  Saturation/1 -> Add/1, Add1/1, Van_inv/1, Mux/1, Relational Operator/1
  Saturation1/1 -> Vbn_inv/1, Relational Operator1/1, Add/2, Add2/1
  Add/1 -> Gain/1
  Add1/1 -> abcs2dqs/1(as)
  Gain/1 -> Add3/2, Add2/2, Add1/2
  Add3/1 -> abcs2dqs/3(cs)
  Saturation2/1 -> Add3/1, Add/3, Vcn_inv/1, Relational Operator2/1
  abcs2dqs/1(ds) -> Vds_stator/1
  abcs2dqs/2(qs) -> Vqs_stator/1
  Mux/1 -> Scope4/1

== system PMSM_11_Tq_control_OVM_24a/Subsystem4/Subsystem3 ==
  In1 : Inport
  In2 : Inport  Port=2
  Add : Sum
  Math Function : Math  Operator=square
  Product : Product
  Product1 : Product
  Out1 : Outport
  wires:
  In1/1 -> Product/2, Product/1
  Product/1 -> Add/1
  Product1/1 -> Add/2
  Add/1 -> Math Function/1
  In2/1 -> Product1/2, Product1/1
  Math Function/1 -> Out1/1

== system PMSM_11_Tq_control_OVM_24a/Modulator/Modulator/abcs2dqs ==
  as : Inport
  bs : Inport  Port=2
  cs : Inport  Port=3
  Gain : Gain  Gain=1/sqrt(3)
  Subtract : Sum  Inputs=+-
  ds : Outport  VectorParamsAs1DForOutWhenUnconnected=off
  qs : Outport  Port=2  VectorParamsAs1DForOutWhenUnconnected=off
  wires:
  Subtract/1 -> Gain/1
  Gain/1 -> qs/1
  bs/1 -> Subtract/1
  cs/1 -> Subtract/2
  as/1 -> ds/1
